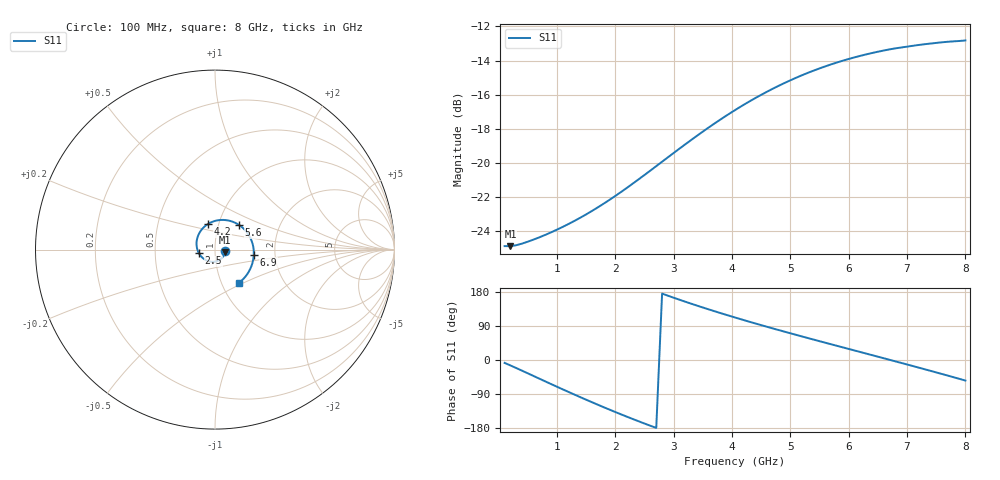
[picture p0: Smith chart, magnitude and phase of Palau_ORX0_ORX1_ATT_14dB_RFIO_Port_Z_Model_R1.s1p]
! Created Fri Oct  9 14:28:29 2020
! Palau ORX0/ORX1 RFIO Port Impedance Model.
! Attenuation  : 14 dB.
! Revision		: R1.
! Impedance Mode 	: Balanced Differential-Mode.
! Impedance Format 	: Series Equivalent Differential Impedance (SEDZ).
# hz S ma R 100
! 1 Port Network Data from SP1.SP block
! freq  magS11  angS11
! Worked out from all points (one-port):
!   80 points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, 100 MHz to 8 GHz, reference 100 ohm
!   lowest |S11| = -24.9 dB at 200 MHz (marker M1), VSWR 1.12, Z = 112 - j3.16 ohm
!   |S11| at or under -10 dB: start of sweep to end of sweep
!   S11 on the Smith chart (normalised r, x): 100 MHz: 1.12, -0.02; 2.5 GHz: 0.83, -0.03; 4.2 GHz: 0.89, +0.26; 5.6 GHz: 1.25, +0.36; 6.9 GHz: 1.55, -0.10; 8 GHz: 1.21, -0.47
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1e8  0.05689 -7.7
2e8  0.05686 -14.4
6e8  0.05949 -42.4
1.1e9  0.06483 -77.7
1.4e9  0.06897 -98.2
1.6e9  0.07219 -111.6
1.8e9  0.07583 -124.6
2.1e9  0.08211 -143.6
2.5e9  0.09208 -167.7
2.8e9  0.1007 175.2
3.1e9  0.11 158.9
3.3e9  0.1166 148.5
3.6e9  0.1269 133.5
4.1e9  0.1444 109.9
4.2e9  0.1479 105.3
4.5e9  0.1583 92.0
4.7e9  0.165 83.3
5.1e9  0.1777 66.3
5.3e9  0.1836 57.9
5.6e9  0.1919 45.5
5.8e9  0.197 37.3
6.1e9  0.2039 25.1
6.5e9  0.2118 8.7
6.9e9  0.2179 -7.7
7.1e9  0.2205 -16.0
7.5e9  0.2248 -32.8
7.7e9  0.2265 -41.3
8e9  0.2285 -54.2
